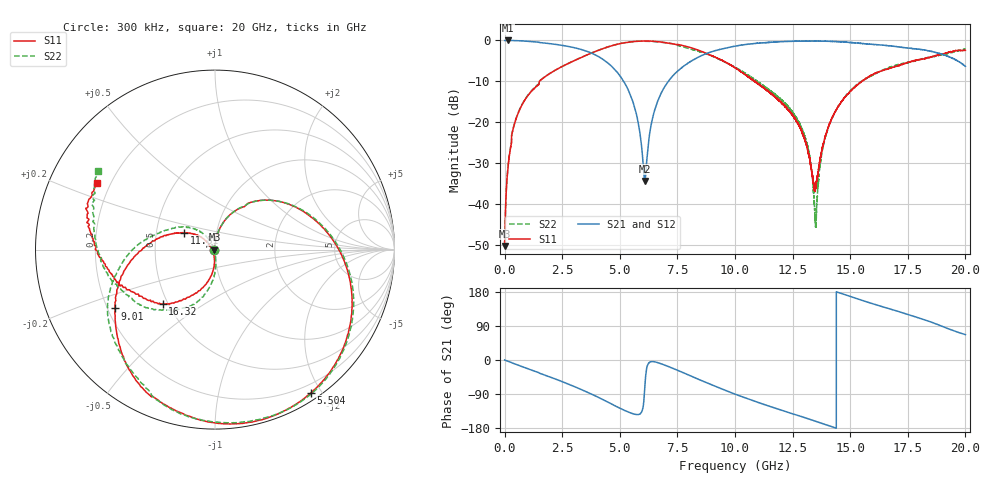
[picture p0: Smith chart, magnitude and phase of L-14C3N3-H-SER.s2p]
!{L-14C3N3}
!Johanson Technology Inc.
!www.johansontechnology.com
!Test Board Conditions:
!Substrate Type  RO4350B
!Substrate Thickness  20 mil
!Substrate Dk  3.66
!TL Type: GCPW
!TL Trace Width  36 mil
!TL Gap  12 mil
!Electrode orientation  Horizontal
!DUT TOPOLOGY	SERIES
!Mounting Pad LxW  26x36 mil
! Created Sun Jun 20 12:56:19 2021
# hz S ma R 50
! 2 Port Network Data from SP1.SP block
! freq  magS11  angS11  magS21  angS21  magS12  angS12  magS22  angS22
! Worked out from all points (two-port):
!   20001 points, 300 kHz to 20 GHz, reference 50 ohm
!   highest |S21| = -0.02 dB at 130.3 MHz (marker M1); lowest = -34.3 dB at 6.088 GHz (marker M2)
!   |S21| within 3 dB of the highest: start of sweep to 3.734 GHz; 8.859 GHz to 18.75 GHz (9.891 GHz wide, 71.7 % of centre)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
!   lowest |S11| = -50.2 dB at 1.3 MHz (marker M3), VSWR 1.01, Z = 49.7 + j0.00718 ohm
!   |S11| at or under -10 dB: start of sweep to 1.504 GHz; 10.84857 GHz to 10.85092 GHz (2.356 MHz wide, 0.0217 % of centre); 10.86 GHz to 15.5 GHz (4.645 GHz wide, 35.2 % of centre)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
!   |S22| runs from -50.2 to -0.2 dB; largest |S21 - S12| = 0.017
!   S11 on the Smith chart (normalised r, x): 300 kHz: 0.99, +0.00; 5.504 GHz: 0.09, -1.87; 9.01 GHz: 0.23, -0.26; 11.81 GHz: 0.70, +0.14; 16.32 GHz: 0.47, -0.34; 20 GHz: 0.15, +0.26
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300000  0.003508 177.8  0.9972 0.0  0.9959 -0.0  0.003219 176.5
1300000  0.003092 178.7  0.997 -0.0  0.9969 -0.1  0.003081 173.4
1.303e8  0.02523 91.2  0.9983 -3.0  0.9974 -2.9  0.02566 91.1
4.003e8  0.08936 80.9  0.9953 -9.3  0.9951 -9.3  0.09073 80.6
8.753e8  0.1866 69.8  0.981 -20.1  0.9803 -20.1  0.1887 69.3
3.3343e9  0.62 10.5  0.7731 -78.1  0.7739 -78.1  0.6213 11.4
4.5123e9  0.8369 -24.4  0.5212 -112.1  0.5224 -112.0  0.839 -23.1
5.5043e9  0.9611 -56.2  0.2003 -140.4  0.2005 -140.4  0.9628 -54.9
6.0883e9  0.9828 -74.1  0.01922 -70.5  0.01954 -70.3  0.9782 -73.2
6.6673e9  0.9641 -90.9  0.1883 -7.4  0.1885 -7.1  0.9589 -91.0
9.0103e9  0.6463 -149.5  0.7299 -65.9  0.7315 -66.2  0.6447 -156.6
1.00003e10  0.4647 -173.3  0.8499 -90.0  0.8525 -90.1  0.4701 -178.6
1.18143e10  0.1953 151.0  0.9582 -128.5  0.9567 -128.6  0.2106 143.6
1.28483e10  0.08322 136.1  0.9783 -148.7  0.9791 -148.7  0.09034 123.8
1.33343e10  0.02468 153.0  0.983 -158.3  0.9824 -158.4  0.02507 124.7
1.35063e10  0.0163 -141.2  0.9828 -161.8  0.9802 -161.8  0.005797 -154.0
1.38163e10  0.05288 -93.6  0.9799 -168.1  0.9796 -168.1  0.049 -84.9
1.42653e10  0.121 -95.7  0.9693 -177.3  0.9711 -177.3  0.1207 -89.8
1.63223e10  0.421 -134.0  0.8799 142.0  0.875 142.1  0.4228 -127.2
1.66673e10  0.4482 -140.3  0.8606 135.9  0.8487 135.7  0.4659 -133.6
1.86333e10  0.6411 -176.0  0.7218 97.4  0.7187 97.7  0.6383 -175.1
2e10  0.7547 150.7  0.4817 67.0  0.4726 67.2  0.7861 145.7
